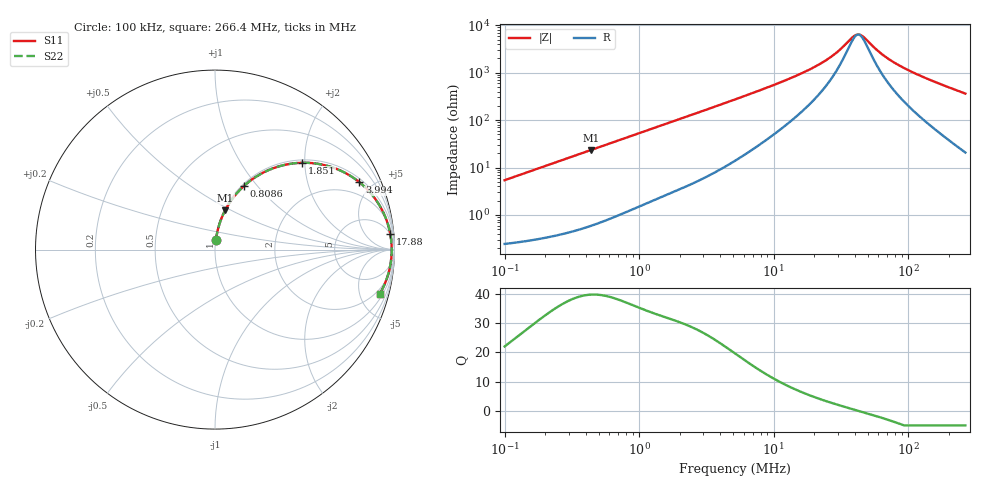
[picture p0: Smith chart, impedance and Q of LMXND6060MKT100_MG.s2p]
! LMXND6060MKT100_MG  S-PARAMETER MODEL  ( General Type )
! Model Generated by TAIYO YUDEN Corporation (https://www.yuden.co.jp/en/)
! Version 1.0
! TAIYO YUDEN Control No. 191025NI43SB-FBB
! Copyright(c) 2019 TAIYO YUDEN CO.,LTD. All Rights Reserved.
! Product Description (link to TY-COMPAS)
! https://ds.yuden.co.jp/TYCOMPAS/or/detail?pn=LMXND6060MKT100MMG&u=M
! Products Name : Inductors
! Characteristics :
!  Inductance : 10 uH , SRF(min) : 22 MHz , DC Resistance(max) : 0.24 Ohm
!  Rated Current : Saturation :1000 mA , Temp Rise : 1200 mA (40 degC)
!  Case Size : 6.0 x 6.0 / 0.236 x 0.236 [mm/inch] , Thickness : 1.2 / 0.047 [mm/inch]
!  (Conditions: Temperature = 25 degC , DC Bias Current/Voltage = 0A / 0V)
! External Node Assignments :
!  1  o---GGG---o  2
! GND o---------o GND
! Frequency Range : 0.1MHz  -  266.375554MHz  [ 402 STEP ]
# MHz S RI R 50
! Freq[MHz].  S11 Real  S11 Imag  S21 Real  S21 Imag  S12 Real  S12 Imag  S22 Real  S22 Imag
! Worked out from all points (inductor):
!   401 points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, 100 kHz to 266.4 MHz, reference 50 ohm
!   read as one part in series: L = 8.59 uH near 104 kHz
!   highest Q = 39.7 at 438.8 kHz (marker M1), where L = 8.51 uH
!   self-resonance near 42.56 MHz
!   S11 on the Smith chart (normalised r, x): 100 kHz: 1.00, +0.11; 808.6 kHz: 1.02, +0.86; 1.851 MHz: 1.06, +1.95; 3.994 MHz: 1.18, +4.20; 17.88 MHz: 5, +22; 266.4 MHz: 1.41, -7.23
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0.1  0.00534 0.0536  0.9947 -0.0536  0.9947 -0.0536  0.00534 0.0536
0.203374  0.015 0.1074  0.985 -0.1074  0.985 -0.1074  0.015 0.1074
0.374775  0.0432 0.191  0.9568 -0.191  0.9568 -0.191  0.0432 0.191
0.438814  0.0572 0.22  0.9428 -0.22  0.9428 -0.22  0.0572 0.22
0.808641  0.1627 0.3558  0.8373 -0.3558  0.8373 -0.3558  0.1627 0.3558
1.404561  0.3588 0.4646  0.6412 -0.4646  0.6412 -0.4646  0.3588 0.4646
1.851113  0.4872 0.4839  0.5128 -0.4839  0.5128 -0.4839  0.4872 0.4839
2.639856  0.6524 0.4587  0.3476 -0.4587  0.3476 -0.4587  0.6524 0.4587
3.994097  0.8049 0.3752  0.1951 -0.3752  0.1951 -0.3752  0.8049 0.3752
5.26394  0.8733 0.3078  0.1267 -0.3078  0.1267 -0.3078  0.8733 0.3078
10.49643  0.9565 0.1618  0.0435 -0.1618  0.0435 -0.1618  0.9565 0.1618
17.87568  0.9769 0.0852  0.0231 -0.0852  0.0231 -0.0852  0.9769 0.0852
19.34272  0.9785 0.076  0.0215 -0.076  0.0215 -0.076  0.9785 0.076
27.04587  0.9828 0.041  0.0172 -0.041  0.0172 -0.041  0.9828 0.041
38.56988  0.9845 0.00863  0.0155 -0.00863  0.0155 -0.00863  0.9845 0.00863
41.73527  0.9846 0.0017  0.0154 -0.0017  0.0154 -0.0017  0.9846 0.0017
46.05978  0.9845 -0.00694  0.0155 0.00694  0.0155 0.00694  0.9845 -0.00694
59.51829  0.9837 -0.0299  0.0163 0.0299  0.0163 0.0299  0.9837 -0.0299
72.49162  0.9822 -0.0488  0.0178 0.0488  0.0178 0.0488  0.9822 -0.0488
91.84439  0.979 -0.0738  0.021 0.0738  0.021 0.0738  0.979 -0.0738
123.455  0.972 -0.1105  0.028 0.1105  0.028 0.1105  0.972 -0.1105
266.3756  0.917 -0.2488  0.083 0.2488  0.083 0.2488  0.917 -0.2488
